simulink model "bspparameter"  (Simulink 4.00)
settings: Solver=ode45  SolverMode=SingleTasking  StartTime=0.0  StopTime=500.0  FixedStep=0.01  RelTol=1e-3
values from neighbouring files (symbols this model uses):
  Konst = 1.15    [bspparameter_ini.m]
  verst = 10    [bspparameter_ini.m]
libraries: simulink3 x1

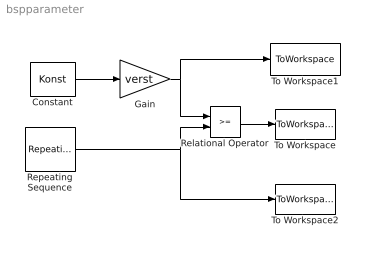
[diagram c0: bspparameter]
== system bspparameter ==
  Constant : Constant  Value=Konst
  Gain : Gain  Gain=verst  Multiplication=Element-wise(K.*u)  SaturateOnIntegerOverflow=on
  Relational Operator : RelationalOperator  Operator=>=
  Repeating Sequence : simulink3/Sources/Repeating Sequence  rep_seq_t=zeit  rep_seq_y=wiederhol
  To Workspace : ToWorkspace  VariableName=erg  SampleTime=-1  SaveFormat=Array
  To Workspace1 : ToWorkspace  VariableName=verst_Konst  SampleTime=-1  SaveFormat=Array
  To Workspace2 : ToWorkspace  VariableName=repeat  SampleTime=-1  SaveFormat=Array
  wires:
  Relational Operator/1 -> To Workspace/1
  Repeating Sequence/1 -> Relational Operator/2, To Workspace2/1
  Constant/1 -> Gain/1
  Gain/1 -> Relational Operator/1, To Workspace1/1
